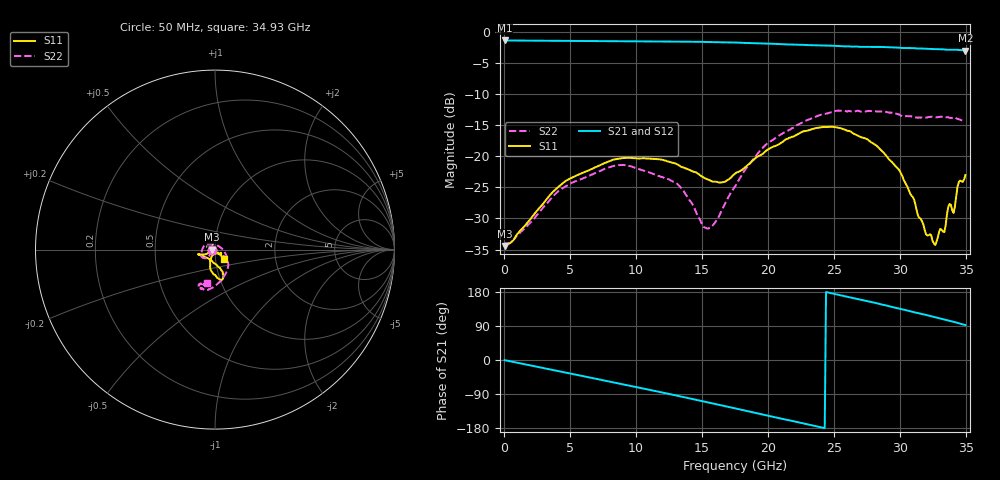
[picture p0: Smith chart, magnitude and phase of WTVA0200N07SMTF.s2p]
! 50 ohm 2-Port S-parameters measured by Modelithics Inc support@modelithics.com  Tampa, FL USA 813-866-6335 (February 2024)
! Smiths Interconnect,  2dB P/N: WTVA0200N07SMTF, Temperature: 75 C
! Board: 10 mil Rogers 4350B, Mounting Pad Dimensions: Length: 15 mils, Width: 25 mils, Gap: 40 mils.
# Hz S RI R 50
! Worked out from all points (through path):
!   352 points, 50 MHz to 34.93 GHz, reference 50 ohm
!   highest |S21| = -1.40 dB at 50 MHz (marker M1); lowest = -3.0 dB at 34.93 GHz (marker M2)
!   group delay of S21, straight-line fit = 21.1 ps
!   lowest |S11| = -34.4 dB at 50 MHz (marker M3), VSWR 1.04, Z = 48.1 + j0.0482 ohm
!   |S11| at or under -10 dB: start of sweep to end of sweep
!   |S22| runs from -34.4 to -12.7 dB; largest |S21 - S12| = 0.0098
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5e7  -0.019 0.0005  0.8511 -0.00498  0.8502 -0.00483  -0.019 -0.000432
3.6825e9  -0.0459 -0.0234  0.7592 -0.3735  0.7581 -0.374  -0.0316 -0.0353
5.8715e9  -0.0676 -0.0274  0.6285 -0.5614  0.6278 -0.561  -0.0452 -0.0476
8.8565e9  -0.0925 -0.026  0.3797 -0.7467  0.3775 -0.7467  -0.0759 -0.0386
1.1742e10  -0.0909 -0.0271  0.0865 -0.8296  0.0846 -0.8289  -0.0692 0.00585
1.3334e10  -0.0774 -0.0309  -0.0847 -0.8285  -0.0867 -0.8274  -0.0481 0.0304
1.54235e10  -0.0472 -0.0449  -0.3071 -0.769  -0.3102 -0.7666  0.00936 0.0245
1.6518e10  -0.0272 -0.0554  -0.413 -0.7115  -0.4143 -0.7098  0.0366 0.00796
1.7513e10  -0.0103 -0.0722  -0.5021 -0.647  -0.5024 -0.6456  0.0549 -0.0172
1.98015e10  0.0295 -0.1058  -0.6636 -0.4554  -0.6632 -0.4543  0.0722 -0.0998
2.33835e10  0.0455 -0.1595  -0.7742 -0.0978  -0.7734 -0.0975  -0.00278 -0.2035
2.61695e10  0.0147 -0.1585  -0.7379 0.1919  -0.7365 0.1939  -0.0706 -0.2198
2.91545e10  -0.0269 -0.0903  -0.5903 0.4638  -0.5849 0.4689  -0.0899 -0.2054
2.99505e10  -0.0276 -0.0711  -0.5263 0.5262  -0.5227 0.5285  -0.0906 -0.1953
3.19405e10  -0.00329 -0.0234  -0.3514 0.6404  -0.3485 0.6407  -0.0709 -0.1915
3.2637e10  0.00598 -0.0184  -0.2837 0.6677  -0.2793 0.6684  -0.0686 -0.1943
3.3035e10  0.0167 -0.0201  -0.2422 0.6811  -0.2357 0.6822  -0.0655 -0.1972
3.33335e10  0.017 -0.0178  -0.2089 0.6901  -0.2044 0.6905  -0.0669 -0.1953
3.37315e10  0.0337 -0.0239  -0.1673 0.6974  -0.1612 0.6979  -0.0621 -0.1935
3.403e10  0.0291 -0.0195  -0.1376 0.7032  -0.1308 0.7036  -0.06 -0.1962
3.4428e10  0.0479 -0.0396  -0.085 0.7089  -0.083 0.7081  -0.0561 -0.1902
3.49255e10  0.0501 -0.0498  -0.029 0.7049  -0.0281 0.7038  -0.0461 -0.1875
